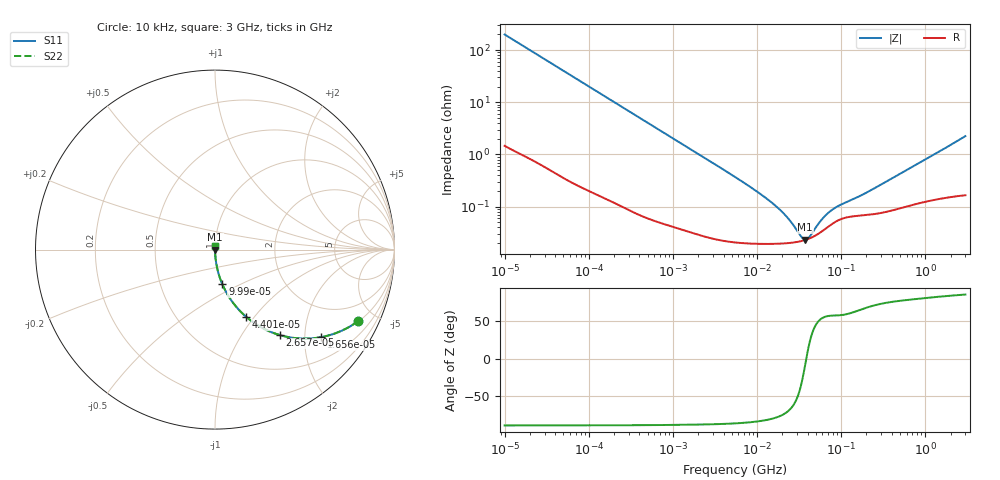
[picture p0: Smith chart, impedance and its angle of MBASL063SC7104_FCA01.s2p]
! MBASL063SC7104_FCA01  S-PARAMETER MODEL  ( Standard Model )
! Model Generated by TAIYO YUDEN Corporation (http://www.ty-top.com)
! Version 1.0
! TAIYO YUDEN Control No. 231201
! Copyright(c) 2023 TAIYO YUDEN CO.,LTD. All Rights Reserved.
! Product Description (link to TY-COMPAS)
! https://ds.yuden.co.jp/TYCOMPAS/or/detail?pn=MBASL063SC7104KFCA01&u=M
! Products Name : Multilayer Ceramic Capacitors
! Characteristics :
!  Capacitance : 0.1 [uF] , Rated Voltage : 10 [V] , TCC : X7S
!  Case Size : 0.6 x 0.3 / 0.024 x 0.012 [mm/inch] , Thickness : 0.3 / 0.012 [mm/inch]
!  (Conditions: Temperature = 25 [degC] , DC Bias Voltage = 0 [V])
! External Node Assignments :
!  1  o---| |---o  2
! GND o---------o GND
! Frequency Range : 10kHz  -  3GHz  [ 401 STEP ]
# MHZ S RI R 50
! Freq[MHz].  S11 Real  S11 Imag  S21 Real  S21 Imag  S12 Real  S12 Imag  S22 Real  S22 Imag
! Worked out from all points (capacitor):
!   401 points, 10 kHz to 3 GHz, reference 50 ohm
!   read as one part in series: C = 79.9 nF near 10.65 kHz
!   lowest |Z| = 23.2 mohm at 37.48 MHz (marker M1)
!   series resonance near 38.58 MHz, so ESL is about 210 pH
!   S11 on the Smith chart (normalised r, x): 10 kHz: 1.03, -3.98; 16.56 kHz: 1.02, -2.41; 26.57 kHz: 1.01, -1.50; 44.01 kHz: 1.01, -0.91; 99.9 kHz: 1.00, -0.40; 3 GHz: 1.00, +0.04
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0.01  0.7967 -0.3988  0.2033 0.3988  0.2033 0.3988  0.7967 -0.3988
0.016561  0.5912 -0.4876  0.4088 0.4876  0.4088 0.4876  0.5912 -0.4876
0.026575  0.3627 -0.4765  0.6373 0.4765  0.6373 0.4765  0.3627 -0.4765
0.044011  0.1741 -0.3748  0.8259 0.3748  0.8259 0.3748  0.1741 -0.3748
0.058452  0.1077 -0.3056  0.8923 0.3056  0.8923 0.3056  0.1077 -0.3056
0.082683  0.0578 -0.2287  0.9422 0.2287  0.9422 0.2287  0.0578 -0.2287
0.099902  0.0408 -0.1929  0.9592 0.1929  0.9592 0.1929  0.0408 -0.1929
0.234035  0.00845 -0.0857  0.9916 0.0857  0.9916 0.0857  0.00845 -0.0857
0.683653  0.00138 -0.0297  0.9986 0.0297  0.9986 0.0297  0.00138 -0.0297
5.477226  0.00022 -0.0037  0.9998 0.0037  0.9998 0.0037  0.00022 -0.0037
10.95979  0.000196 -0.00174  0.9998 0.00174  0.9998 0.00174  0.000196 -0.00174
17.04125  0.000195 -0.000983  0.9998 0.000983  0.9998 0.000983  0.000195 -0.000983
24.10585  0.000201 -0.000528  0.9998 0.000528  0.9998 0.000528  0.000201 -0.000528
34.09912  0.00022 -0.000134  0.9998 0.000134  0.9998 0.000134  0.00022 -0.000134
37.4819  0.00023 -3.12e-05  0.9998 3.12e-05  0.9998 3.12e-05  0.00023 -3.12e-05
41.20027  0.000242 7.15e-05  0.9998 -7.15e-05  0.9998 -7.15e-05  0.000242 7.15e-05
45.28751  0.000259 0.000174  0.9997 -0.000174  0.9997 -0.000174  0.000259 0.000174
60.14696  0.000343 0.00048  0.9997 -0.00048  0.9997 -0.00048  0.000343 0.00048
79.88199  0.000478 0.000752  0.9995 -0.000752  0.9995 -0.000752  0.000478 0.000752
193.129  0.000688 0.00166  0.9993 -0.00166  0.9993 -0.00166  0.000688 0.00166
374.4521  0.000829 0.00315  0.9992 -0.00315  0.9992 -0.00315  0.000829 0.00315
3000  0.00215 0.0223  0.9979 -0.0223  0.9979 -0.0223  0.00215 0.0223
